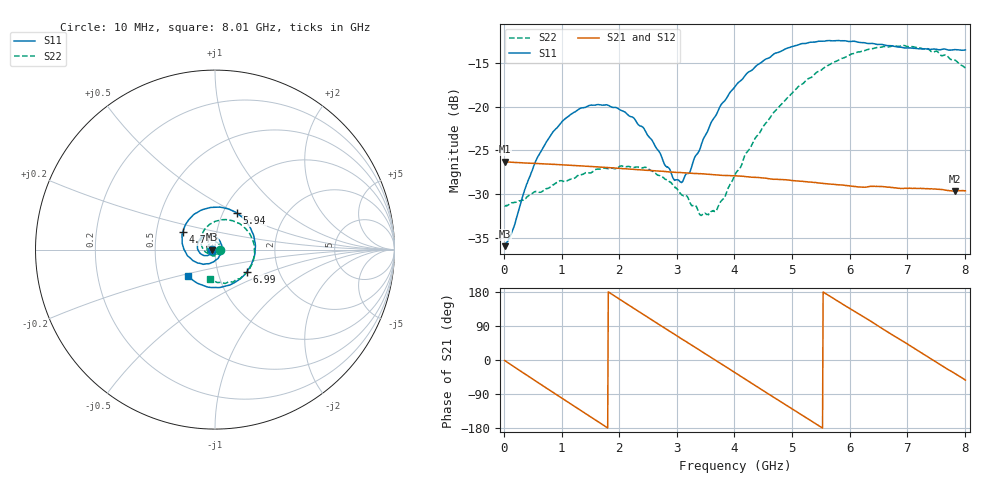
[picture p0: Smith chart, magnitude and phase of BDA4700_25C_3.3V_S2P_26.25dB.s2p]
!Agilent Technologies,E5071B,MY42404982,A.09.10
!Date: Mon Oct 20 18:14:06 2025
!Data & Calibration Information:
!Freq	S11:SOLT2(ON)	S21:SOLT2(ON)	S12:SOLT2(ON)	S22:SOLT2(ON)
# Hz S RI R 50
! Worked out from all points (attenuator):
!   801 points, 10 MHz to 8.01 GHz, reference 50 ohm
!   highest |S21| = -26.31 dB at 10 MHz (marker M1); lowest = -29.7 dB at 7.83 GHz (marker M2)
!   lowest |S11| = -35.9 dB at 10 MHz (marker M3), VSWR 1.03, Z = 48.4 - j0.11 ohm
!   |S11| at or under -10 dB: start of sweep to end of sweep
!   |S22| runs from -32.4 to -13.0 dB; largest |S21 - S12| = 0.00056
!   S11 on the Smith chart (normalised r, x): 10 MHz: 0.97, -0.00; 4.77 GHz: 0.68, +0.14; 5.94 GHz: 1.16, +0.50; 6.99 GHz: 1.38, -0.36; 8.01 GHz: 0.71, -0.22
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1e7  -0.0159 -0.00113  0.0484 -0.000996  0.0483 -0.00108  0.0271 -0.000811
1.5e8  -0.017 -0.00994  0.0462 -0.0128  0.0463 -0.0128  0.0273 -0.0073
6e8  -0.0406 -0.0333  0.0233 -0.0412  0.0232 -0.0411  0.0132 -0.0297
1.01e9  -0.0787 -0.0243  -0.00913 -0.0456  -0.00909 -0.0456  -0.0152 -0.0345
1.35e9  -0.098 0.0074  -0.0324 -0.0324  -0.0324 -0.0324  -0.0365 -0.0182
2.08e9  -0.0495 0.0798  -0.0394 0.0199  -0.0395 0.0199  -0.0302 0.0338
2.68e9  0.0266 0.0493  -0.00362 0.0427  -0.00365 0.0426  0.0129 0.0384
2.95e9  0.0372 0.00891  0.0153 0.0393  0.0152 0.0392  0.0258 0.0238
3.09e9  0.0344 -0.0135  0.024 0.0344  0.0237 0.0345  0.0286 0.0127
3.41e9  0.00387 -0.0582  0.0377 0.0172  0.0376 0.0172  0.0213 -0.0111
3.54e9  -0.016 -0.0712  0.0402 0.00849  0.0402 0.00845  0.0141 -0.0197
3.69e9  -0.0446 -0.0788  0.0406 -0.00174  0.0407 -0.00184  0.00155 -0.0255
4.01e9  -0.1111 -0.0673  0.0336 -0.0221  0.0337 -0.022  -0.0312 -0.0261
4.77e9  -0.1788 0.0986  -0.011 -0.0368  -0.0108 -0.0368  -0.0783 0.0609
5.35e9  -0.0653 0.2238  -0.0353 -0.0111  -0.0352 -0.0113  -0.016 0.1471
5.94e9  0.122 0.2032  -0.0277 0.0221  -0.0278 0.0219  0.1169 0.1529
6.37e9  0.212 0.0877  -0.00732 0.0342  -0.00737 0.034  0.1975 0.0801
6.68e9  0.2215 -0.0225  0.0107 0.033  0.0107 0.033  0.2192 0.00011
6.99e9  0.1768 -0.1239  0.0248 0.0235  0.0249 0.0234  0.2048 -0.0827
7.44e9  0.0401 -0.2088  0.0339 0.000339  0.0339 0.000287  0.116 -0.1683
7.83e9  -0.0975 -0.1877  0.0267 -0.0192  0.0267 -0.0192  0.0135 -0.1834
8.01e9  -0.149 -0.149  0.0199 -0.0264  0.0201 -0.0264  -0.0304 -0.1635
